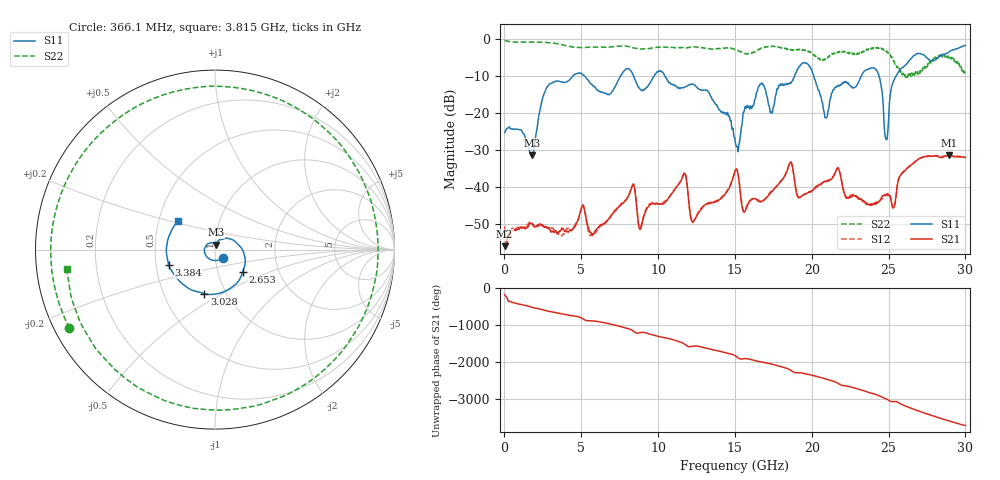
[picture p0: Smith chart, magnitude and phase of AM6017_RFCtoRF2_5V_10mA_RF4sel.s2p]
!Agilent Technologies,E8364B,MY43040894,A.07.50.67
!Agilent E8364B: A.07.50.67
!Date: Tuesday, August 21, 2018 13:37:41
!Correction: S11(Full 2 Port(1,2))
!S21(Full 2 Port(1,2))
!S12(Full 2 Port(1,2))
!S22(Full 2 Port(1,2))
!S2P File: Measurements: S11, S21, S12, S22:
# Hz S  dB  R 50
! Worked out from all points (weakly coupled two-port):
!   1601 points, 10 MHz to 30 GHz, reference 50 ohm
!   highest |S21| = -31.40 dB at 28.93 GHz (marker M1); lowest = -55.9 dB at 10 MHz (marker M2)
!   lowest |S11| = -31.3 dB at 1.772 GHz (marker M3), VSWR 1.06, Z = 50.3 + j2.7 ohm
!   |S11| at or under -10 dB: start of sweep to 4.447 GHz; 10.44 GHz to 18.88 GHz (8.444 GHz wide, 57.6 % of centre); 20.14 GHz to 23.23 GHz (3.093 GHz wide, 14.3 % of centre)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
!   |S22| runs from -10.3 to -0.4 dB; largest |S21 - S12| = 0.0045
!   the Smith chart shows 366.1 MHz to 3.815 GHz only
!   S11 on the Smith chart (normalised r, x): 366.1 MHz: 1.08, -0.10; 2.653 GHz: 1.32, -0.34; 3.028 GHz: 0.79, -0.41; 3.384 GHz: 0.58, -0.11; 3.815 GHz: 0.63, +0.22
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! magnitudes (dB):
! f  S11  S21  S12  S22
! 10 MHz  -25.3  -55.9  -50.5  -0.4
! 366.1 MHz  -24.0  -52.4  -52.1  -0.7
! 1.772 GHz  -31.3  -49.8  -49.8  -0.8
! 2.653 GHz  -14.1  -50.6  -50.6  -0.9
! 3.028 GHz  -12.0  -52.0  -51.1  -1.0
! 3.384 GHz  -11.3  -52.1  -52.2  -1.3
! 3.815 GHz  -11.7  -51.1  -52.6  -1.6
! 5.015 GHz  -9.3  -45.5  -45.3  -2.3
! 5.689 GHz  -12.2  -52.6  -52.7  -2.2
! 10.02 GHz  -8.7  -44.6  -44.4  -2.2
! 11.71 GHz  -13.0  -36.2  -36.1  -2.4
! 12.31 GHz  -12.2  -49.1  -49.2  -2.1
! 15.01 GHz  -27.3  -35.7  -35.6  -2.9
! 15.62 GHz  -19.0  -46.6  -46.2  -3.9
! 18.6 GHz  -11.9  -33.3  -33.2  -2.8
! 20.01 GHz  -8.5  -41.0  -40.9  -3.8
! 20.93 GHz  -21.2  -38.3  -38.2  -5.4
! 24.08 GHz  -7.9  -44.5  -44.3  -2.4
! 25.01 GHz  -20.4  -42.2  -41.8  -3.8
! 25.78 GHz  -8.1  -36.7  -36.5  -8.9
! 28.93 GHz  -3.5  -31.4  -31.3  -5.1
! 30 GHz  -1.7  -31.9  -31.9  -9.2
